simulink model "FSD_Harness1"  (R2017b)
settings: Solver=FixedStepDiscrete  StartTime=0.0  StopTime=4  FixedStep=0.01  RelTol=1e-3  EnableMultiTasking=on
undefined symbols (not defined in the file): sigbuilder_block

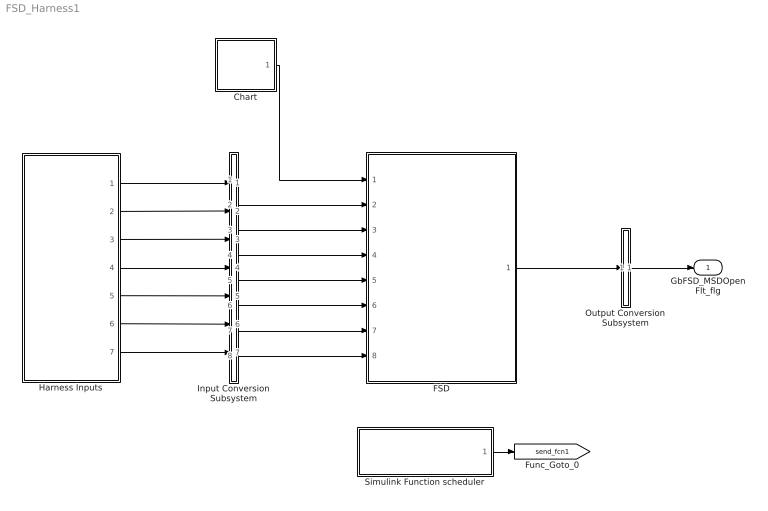
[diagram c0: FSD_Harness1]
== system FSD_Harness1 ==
  Chart : Stateflow chart  TreatAsAtomicUnit=on
  FSD : ModelReference  ModelNameDialog=FSD  SimulationMode=Normal  ModelReferenceVersion='M102C102R103'
  Harness Inputs : Subsystem  Tag=STV Subsys  LoadFcn=sigbuilder_block('load');  StartFcn=sigbuilder_block('start');  StopFcn=sigbuilder_block('stop');  ClipboardFcn=sigbuilder_block('clipboard');  mask(Sigbuilder block){tuvar=[0:10]}
      mask init:
      | if ~strcmp(get_param(bdroot(gcb),'SimulationStatus'),'stopped'),tuvar = sigbuilder_block('maskInit'); end
  Input Conversion Subsystem : Subsystem  Tag=__SLT_ICS__  Description=Signal spec. and routing
  Output Conversion Subsystem : Subsystem  Tag=__SLT_OCS__  Description=Signal spec. and routing
  Simulink Function scheduler : Test Sequence  Tag=__SLT_FCN_CALL__  TreatAsAtomicUnit=on
  GbFSD_MSDOpenFlt_flg : Outport  OutDataTypeStr=boolean  PortDimensions=[1]
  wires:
  Harness Inputs/1(GbHVL_HvilLFlt_flg) -> Input Conversion Subsystem/1(Inport_1)
  Harness Inputs/2(GbHDP_PackVoltVld_flg) -> Input Conversion Subsystem/2(Inport_2)
  Harness Inputs/3(GcHDP_PackVolt_V) -> Input Conversion Subsystem/3(Inport_3)
  Harness Inputs/4(GcCDP_SumCellVolt_V) -> Input Conversion Subsystem/4(Inport_4)
  Harness Inputs/5(GbCDP_SumCellVoltVld_flg) -> Input Conversion Subsystem/5(Inport_5)
  Harness Inputs/6(GbHDP_FuseVoltVld_flg) -> Input Conversion Subsystem/6(Inport_6)
  Harness Inputs/7(GcHDP_FuseVolt_V) -> Input Conversion Subsystem/7(Inport_7)
  Output Conversion Subsystem/1(Outport_1) -> GbFSD_MSDOpenFlt_flg/1
  Chart/1(RUN100ms()) -> FSD/1
  Input Conversion Subsystem/2(Outport_2) -> FSD/2
  Input Conversion Subsystem/3(Outport_3) -> FSD/3
  Input Conversion Subsystem/4(Outport_4) -> FSD/4
  Input Conversion Subsystem/5(Outport_5) -> FSD/5
  Input Conversion Subsystem/6(Outport_6) -> FSD/6
  Input Conversion Subsystem/7(Outport_7) -> FSD/7
  Input Conversion Subsystem/8(Outport_8) -> FSD/8
  FSD/1 -> Output Conversion Subsystem/1(Inport_1)
  Simulink Function scheduler/1(FSD_FuseDiag_100ms()) -> [send_fcn1]

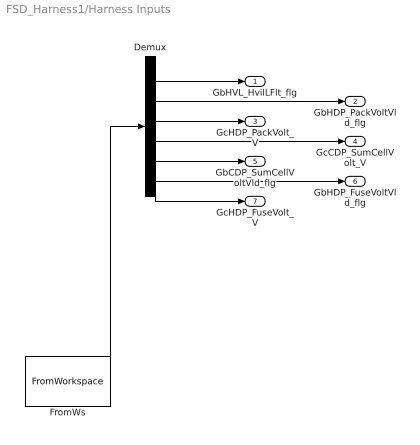
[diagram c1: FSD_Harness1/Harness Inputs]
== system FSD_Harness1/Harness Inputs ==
  Demux : Demux  Tag=STV Demux  Outputs=7
  FromWs : FromWorkspace  Tag=STV FromWs  VariableName=tuvar  SampleTime=0
  GbHVL_HvilLFlt_flg : Outport  Tag=STV Outport
  GbHDP_PackVoltVld_flg : Outport  Tag=STV Outport  Port=2
  GcHDP_PackVolt_V : Outport  Tag=STV Outport  Port=3
  GcCDP_SumCellVolt_V : Outport  Tag=STV Outport  Port=4
  GbCDP_SumCellVoltVld_flg : Outport  Tag=STV Outport  Port=5
  GbHDP_FuseVoltVld_flg : Outport  Tag=STV Outport  Port=6
  GcHDP_FuseVolt_V : Outport  Tag=STV Outport  Port=7
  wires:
  FromWs/1 -> Demux/1
  Demux/1 -> GbHVL_HvilLFlt_flg/1
  Demux/2 -> GbHDP_PackVoltVld_flg/1
  Demux/3 -> GcHDP_PackVolt_V/1
  Demux/4 -> GcCDP_SumCellVolt_V/1
  Demux/5 -> GbCDP_SumCellVoltVld_flg/1
  Demux/6 -> GbHDP_FuseVoltVld_flg/1
  Demux/7 -> GcHDP_FuseVolt_V/1

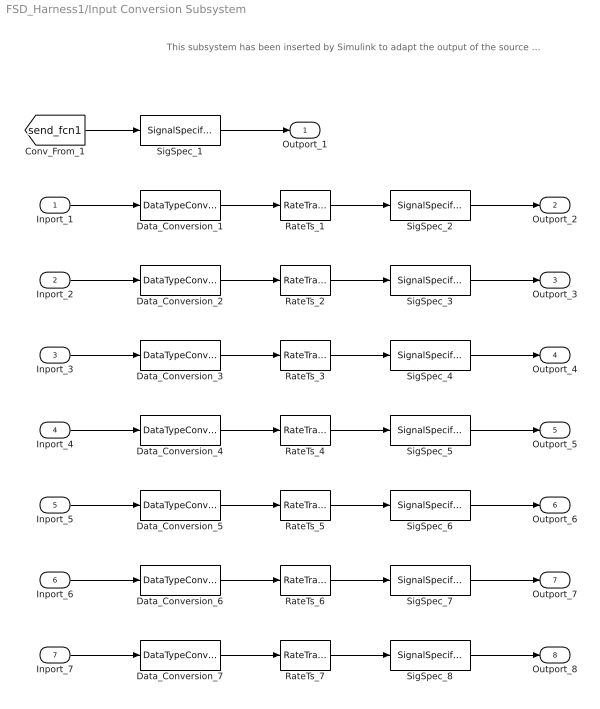
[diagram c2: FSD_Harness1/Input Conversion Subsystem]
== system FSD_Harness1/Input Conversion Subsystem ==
  note: This subsystem has been inserted by Simulink to adapt the output of the source blocks to the interface required by the harnessed component. Modifying the contents of this subsystem may result in compilation and simulation failure.
  Inport_1 : Inport
  Inport_2 : Inport  Port=2
  Inport_3 : Inport  Port=3
  Inport_4 : Inport  Port=4
  Inport_5 : Inport  Port=5
  Inport_6 : Inport  Port=6
  Inport_7 : Inport  Port=7
  Data_Conversion_{1..2,5..6} (4 alike) : DataTypeConversion  OutDataTypeStr=boolean
  Data_Conversion_3 : DataTypeConversion  OutDataTypeStr=single
  Data_Conversion_4 : DataTypeConversion  OutDataTypeStr=single
  Data_Conversion_7 : DataTypeConversion  OutDataTypeStr=single
  RateTs_{1..7} (7 alike) : RateTransition
  SigSpec_1 : SignalSpecification
  SigSpec_{2..3,6..7} (4 alike) : SignalSpecification  OutDataTypeStr=boolean  Unit=flag  Dimensions=[1]
  SigSpec_4 : SignalSpecification  OutDataTypeStr=single  Unit=V  Dimensions=[1]
  SigSpec_5 : SignalSpecification  OutDataTypeStr=single  Unit=V  Dimensions=[1]
  SigSpec_8 : SignalSpecification  OutDataTypeStr=single  Unit=V  Dimensions=[1]
  Outport_1 : Outport
  Outport_2 : Outport  Port=2
  Outport_3 : Outport  Port=3
  Outport_4 : Outport  Port=4
  Outport_5 : Outport  Port=5
  Outport_6 : Outport  Port=6
  Outport_7 : Outport  Port=7
  Outport_8 : Outport  Port=8
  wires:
  SigSpec_1/1 -> Outport_1/1
  [send_fcn1] -> SigSpec_1/1
  SigSpec_2/1 -> Outport_2/1
  RateTs_1/1 -> SigSpec_2/1
  Data_Conversion_1/1 -> RateTs_1/1
  Inport_1/1 -> Data_Conversion_1/1
  SigSpec_3/1 -> Outport_3/1
  RateTs_2/1 -> SigSpec_3/1
  Data_Conversion_2/1 -> RateTs_2/1
  Inport_2/1 -> Data_Conversion_2/1
  SigSpec_4/1 -> Outport_4/1
  RateTs_3/1 -> SigSpec_4/1
  Data_Conversion_3/1 -> RateTs_3/1
  Inport_3/1 -> Data_Conversion_3/1
  SigSpec_5/1 -> Outport_5/1
  RateTs_4/1 -> SigSpec_5/1
  Data_Conversion_4/1 -> RateTs_4/1
  Inport_4/1 -> Data_Conversion_4/1
  SigSpec_6/1 -> Outport_6/1
  RateTs_5/1 -> SigSpec_6/1
  Data_Conversion_5/1 -> RateTs_5/1
  Inport_5/1 -> Data_Conversion_5/1
  SigSpec_7/1 -> Outport_7/1
  RateTs_6/1 -> SigSpec_7/1
  Data_Conversion_6/1 -> RateTs_6/1
  Inport_6/1 -> Data_Conversion_6/1
  SigSpec_8/1 -> Outport_8/1
  RateTs_7/1 -> SigSpec_8/1
  Data_Conversion_7/1 -> RateTs_7/1
  Inport_7/1 -> Data_Conversion_7/1

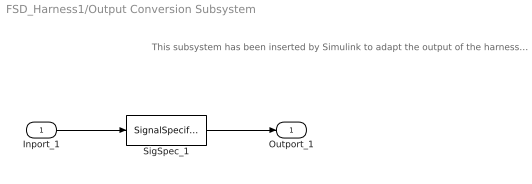
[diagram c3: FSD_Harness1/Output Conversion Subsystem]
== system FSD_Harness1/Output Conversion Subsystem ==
  note: This subsystem has been inserted by Simulink to adapt the output of the harnessed component to the interface required by the sink blocks. Modifying the contents of this subsystem may result in compilation and simulation failure.
  Inport_1 : Inport
  SigSpec_1 : SignalSpecification  OutDataTypeStr=boolean  Unit=flag  Dimensions=[1]
  Outport_1 : Outport
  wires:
  Inport_1/1 -> SigSpec_1/1
  SigSpec_1/1 -> Outport_1/1

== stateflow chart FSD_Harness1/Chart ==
  (default) -> (junction 1)
  (junction 1) -> (junction 3) : {RUN100ms}
  events: output FUNCTION_CALL_EVENT

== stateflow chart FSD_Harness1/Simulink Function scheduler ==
  state Run
  state AsyncFunctionCalls
    % Call Asynchronous FunctionCall Subsystems.
    %
    %% Schedule function-call outputs.
    %% Modify this code to change function-call order.
    send(FSD_FuseDiag_100ms)
  (default) -> Run
  events: output FUNCTION_CALL_EVENT
